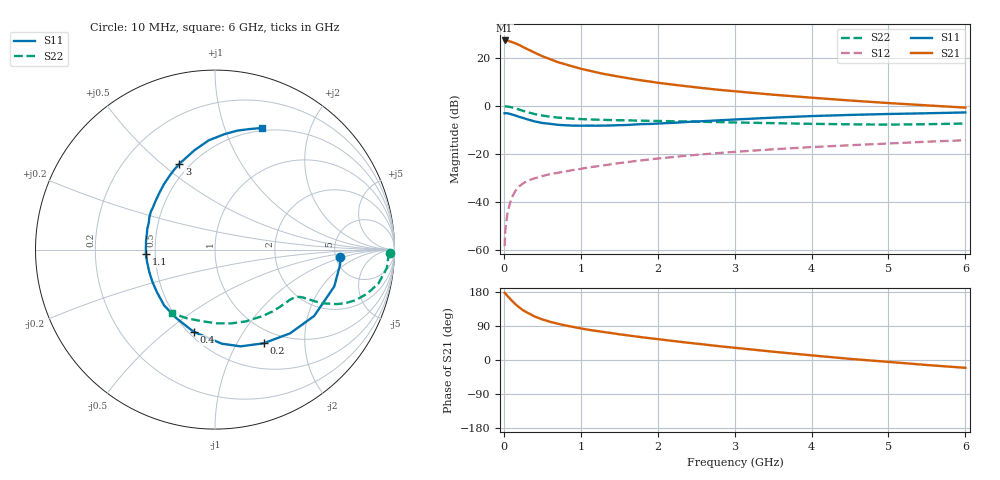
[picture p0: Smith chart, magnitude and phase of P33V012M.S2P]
! SIEMENS Small Signal Semiconductors
! BFP181
! Si NPN RF Bipolar Junction Transistor in SOT143
! VCE = 3 V  IC = 12 mA
! Common Emitter S-Parameters:  March  1996
# GHz  S  MA  R  50
!  f  S11  S21  S12  S22
! GHz  MAG  ANG  MAG  ANG  MAG  ANG  MAG  ANG
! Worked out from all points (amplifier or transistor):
!   36 points, 10 MHz to 6 GHz, reference 50 ohm
!   highest |S21| = 27.2 dB at 10 MHz (marker M1)
!   |S21| within 3 dB of that: start of sweep to 267 MHz
!   unconditionally stable (mu >= 1): 942.7 MHz to end of sweep
!   at 250 MHz: K = 0.39, MSG = 28.4 dB, |S12| = -32.3 dB
!   at 1.4 GHz: K = 1.15, MAG = 16.2 dB, |S12| = -24.3 dB
!   at 6 GHz: K = 1.01, MAG = 6.1 dB, |S12| = -14.3 dB
!   S11 on the Smith chart (normalised r, x): 10 MHz: 5.48, -0.88; 200 MHz: 0.81, -1.30; 400 MHz: 0.53, -0.63; 1.1 GHz: 0.44, -0.03; 3 GHz: 0.44, +0.57; 6 GHz: 0.47, +1.35
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0.01  0.698 -3.4  22.83 177.5  0.0012 92.2  0.973 -1.0
0.02  0.7021 -6.9  22.82 175.5  0.0027 84.6  0.967 -2.3
0.05  0.6953 -17.2  22.55 168.3  0.0064 87.0  0.9629 -6.1
0.1  0.6648 -33.8  21.31 157.5  0.012 74.6  0.9299 -11.7
0.15  0.6264 -48.2  19.91 147.4  0.0169 67.4  0.8821 -16.2
0.2  0.588 -62.6  18.39 138.9  0.0212 63.7  0.8324 -19.8
0.25  0.5576 -75.2  16.66 131.3  0.0242 59.7  0.7841 -22.4
0.3  0.5257 -85.8  15.25 125.5  0.0272 57.4  0.741 -24.2
0.4  0.4735 -104.5  12.74 114.9  0.031 53.5  0.6733 -26.4
0.5  0.438 -119.8  10.74 107.1  0.0344 51.0  0.6258 -27.4
0.6  0.4209 -132.3  9.334 100.9  0.0378 50.4  0.5916 -27.9
0.7  0.4014 -143.5  8.114 95.8  0.0403 50.5  0.5684 -28.4
0.9  0.3869 -160.9  6.538 87.3  0.0461 50.3  0.539 -29.3
1.1  0.3859 -176.1  5.425 79.8  0.0522 50.8  0.52 -30.7
1.5  0.3949 162.7  4.022 67.9  0.0642 51.1  0.4995 -34.5
1.8  0.4156 149.2  3.36 59.9  0.0735 50.2  0.4893 -38.3
2.2  0.4416 134.8  2.748 50.2  0.0859 48.5  0.4764 -43.9
3  0.5178 112.5  2.004 32.3  0.1098 43.5  0.4489 -57.1
3.5  0.5657 101.6  1.7 21.9  0.1243 40.1  0.4352 -66.8
4.5  0.6448 85.4  1.287 3.0  0.1509 32.3  0.4109 -88.9
5.5  0.6982 74.1  1.019 -13.2  0.1788 25.1  0.4136 -112.2
6  0.7264 68.9  0.915 -20.7  0.1919 20.9  0.4271 -124.0
